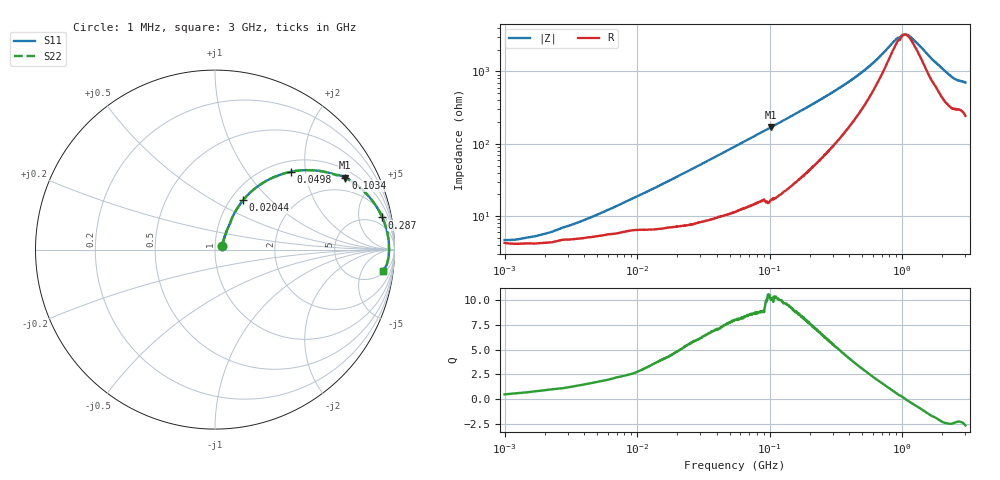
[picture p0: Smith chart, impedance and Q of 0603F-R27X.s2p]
!s-Parameter Generated by FASTRON Sdn. Bhd.
!FASTRON P/N : 0603F-R27X
!Keysight Technologies: E4991B_MY54100416_A.01.15
!Date: Thu Jun 20 13:17:13 2024
!Version  :Rev00  Thu Jun 20 13:17:13 2024
!Data & Calibration Information:
!Freq  S11  S21  S12  S22
!PortZ  Port1:50+j0  Port2:50+j0
!When reading reference impedance value at option line is always used.
! Remarks : This data is being provided solely for informational purposes.
# Hz S dB R 50
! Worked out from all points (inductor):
!   1601 points, 1 MHz to 3 GHz, reference 50 ohm
!   read as one part in series: L = 277 nH near 11.1 MHz
!   highest Q = 10.4 at 102.9 MHz (marker M1), where L = 262 nH
!   self-resonance near 1.053 GHz
!   S11 on the Smith chart (normalised r, x): 1 MHz: 1.08, +0.04; 20.44 MHz: 1.14, +0.70; 49.8 MHz: 1.21, +1.66; 103.4 MHz: 1.34, +3.41; 287 MHz: 3, +10; 3 GHz: 6, -13
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1000000  -27.00 23.4  -0.36 -1.1  -0.36 -1.1  -27.00 23.4
1751453  -25.80 36.3  -0.36 -1.8  -0.36 -1.8  -25.80 36.3
3804036  -21.80 50.8  -0.44 -3.8  -0.44 -3.8  -21.80 50.8
7819618  -17.00 59.2  -0.58 -7.5  -0.58 -7.5  -17.00 59.2
1.447069e7  -12.50 62.0  -0.79 -13.3  -0.79 -13.3  -12.50 62.0
2.043808e7  -9.98 60.3  -1.04 -18.1  -1.04 -18.1  -9.98 60.3
3.158701e7  -7.00 54.8  -1.64 -26.2  -1.64 -26.2  -7.00 54.8
4.980464e7  -4.37 45.8  -2.82 -36.9  -2.82 -36.9  -4.37 45.8
5.504702e7  -3.88 43.5  -3.18 -39.4  -3.18 -39.4  -3.88 43.5
1.028925e8  -1.64 28.9  -6.27 -55.4  -6.27 -55.4  -1.64 28.9
1.034087e8  -1.63 28.8  -6.30 -55.6  -6.30 -55.6  -1.63 28.8
1.445978e8  -1.02 21.7  -8.60 -62.1  -8.60 -62.1  -1.02 21.7
2.083556e8  -0.64 15.3  -11.50 -67.0  -11.50 -67.0  -0.64 15.3
2.870054e8  -0.46 10.9  -14.30 -69.2  -14.30 -69.2  -0.46 10.9
5.102796e8  -0.30 5.2  -20.40 -66.1  -20.40 -66.1  -0.30 5.2
7.925923e8  -0.27 1.9  -27.00 -46.0  -27.00 -46.0  -0.27 1.9
8.982141e8  -0.27 1.0  -29.10 -30.0  -29.10 -30.0  -0.27 1.0
1.007775e9  -0.26 0.3  -30.40 -10.0  -30.40 -10.0  -0.26 0.3
1.10276e9  -0.27 -0.3  -30.30 10.1  -30.30 10.1  -0.27 -0.3
2.278218e9  -0.39 -5.7  -19.40 62.7  -19.40 62.7  -0.39 -5.7
2.556106e9  -0.48 -6.5  -18.20 60.6  -18.20 60.6  -0.48 -6.5
3e9  -0.49 -7.3  -17.40 62.4  -17.40 62.4  -0.49 -7.3
